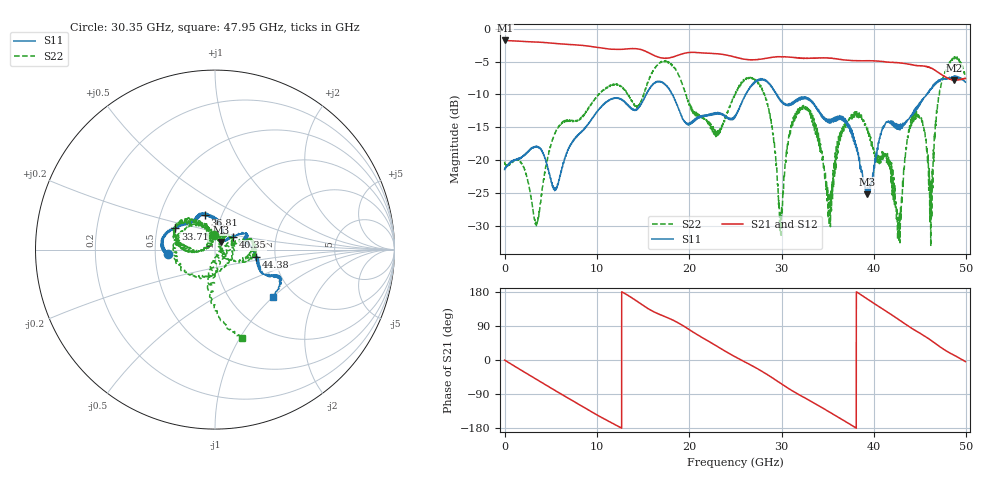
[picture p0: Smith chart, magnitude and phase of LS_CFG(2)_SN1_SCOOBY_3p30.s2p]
!Keysight Technologies,N5245B,MY58422026,A.13.80.08
!Date: Thursday, March 19, 2020 23:27:14
!Correction: S11(Full 2 Port(1,2))
!S21(Full 2 Port(1,2))
!S12(Full 2 Port(1,2))
!S22(Full 2 Port(1,2))
!S2P File: Measurements: S11, S21, S12, S22:
# Hz S DB R 50.0
!freq dBS11 angS11 dBS21 angS21 dBS12 angS12 dBS22 angS22
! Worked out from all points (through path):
!   4991 points, 10 MHz to 49.91 GHz, reference 50 ohm
!   highest |S21| = -1.81 dB at 20 MHz (marker M1); lowest = -7.8 dB at 48.67 GHz (marker M2)
!   group delay of S21, straight-line fit = 39.9 ps
!   lowest |S11| = -25.1 dB at 39.22 GHz (marker M3), VSWR 1.12, Z = 53.5 + j4.54 ohm
!   |S11| at or under -10 dB: start of sweep to 15.34 GHz; 18.16 GHz to 26.09 GHz (7.926 GHz wide, 35.8 % of centre); 29.48 GHz to 45.68 GHz (16.2 GHz wide, 43.1 % of centre)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
!   |S22| runs from -33.0 to -4.3 dB; largest |S21 - S12| = 0.0075
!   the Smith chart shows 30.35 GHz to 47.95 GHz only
!   S11 on the Smith chart (normalised r, x): 30.35 GHz: 0.58, -0.03; 33.71 GHz: 0.62, +0.16; 36.81 GHz: 0.83, +0.33; 40.35 GHz: 1.21, +0.18; 44.38 GHz: 1.58, -0.14; 47.95 GHz: 1.56, -1.00
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1e7  -21.37 -2.3  -1.81 -0.3  -1.80 -0.3  -20.19 1.1
2e7  -21.24 -0.9  -1.81 -0.4  -1.80 -0.4  -20.39 -0.5
3.47e9  -17.87 -51.5  -2.05 -51.1  -2.05 -51.1  -29.64 -53.6
8.33e9  -15.72 -57.1  -2.55 -121.2  -2.54 -121.1  -13.49 -60.0
1.665e10  -8.05 -124.3  -4.33 121.8  -4.32 121.8  -5.39 -160.3
2.496e10  -13.40 -122.3  -4.31 8.7  -4.30 8.8  -10.05 178.5
2.753e10  -7.68 -146.4  -4.67 -24.9  -4.66 -24.8  -8.30 -110.3
2.987e10  -10.99 -175.6  -4.28 -61.1  -4.27 -61.0  -28.16 13.2
3.035e10  -11.58 -174.7  -4.28 -68.7  -4.28 -68.6  -21.50 92.7
3.328e10  -10.98 157.8  -4.50 -110.3  -4.49 -110.0  -13.33 171.3
3.371e10  -12.02 151.9  -4.47 -115.9  -4.46 -115.6  -15.10 171.0
3.518e10  -14.00 123.8  -4.46 -137.3  -4.40 -136.9  -29.80 130.5
3.681e10  -13.99 106.1  -4.76 -160.7  -4.65 -160.8  -14.76 129.9
3.922e10  -25.13 49.7  -4.88 162.1  -4.86 161.8  -15.32 -121.6
4.035e10  -18.24 35.7  -4.93 143.9  -4.93 143.5  -20.09 -35.8
4.16e10  -14.03 26.5  -5.10 124.3  -5.12 124.0  -20.11 61.1
4.273e10  -14.91 15.4  -5.22 106.1  -5.24 105.9  -30.95 -0.0
4.438e10  -12.72 -10.4  -5.58 79.2  -5.61 79.1  -13.17 2.7
4.616e10  -9.15 -24.8  -5.96 52.3  -5.97 52.2  -32.99 -46.2
4.795e10  -7.58 -39.5  -7.52 22.2  -7.54 22.2  -5.81 -73.2
4.867e10  -7.24 -52.0  -7.84 12.8  -7.85 12.8  -4.35 -56.6
4.991e10  -8.14 -52.0  -7.55 -4.1  -7.57 -4.2  -7.35 -25.3
